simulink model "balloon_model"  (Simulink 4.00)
settings: Solver=ode45  StartTime=0.0  StopTime=5000  RelTol=1e-3
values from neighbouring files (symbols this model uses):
  C = V*rho_a*c_a    [balloon_init.m]
  f = f / 10    [balloon_init.m]
  g = 9.80665    [balloon_init.m]
  m = input('Inserire le prime due cifre (esclusi zeri) del proprio numero di matricola:\n\n')    [balloon_init.m]
  rho_a = 1.2928    [balloon_init.m]
  Ta = 20+273.15    (= 293.15)    [balloon_init.m]
  theta_t = theta_t/50    [balloon_init.m]
  V = V*m*2    [balloon_init.m]
  x1_0 = x1_d    [balloon_init.m]
  x2_0 = 100    [balloon_init.m]
  x3_0 = 0    [balloon_init.m]

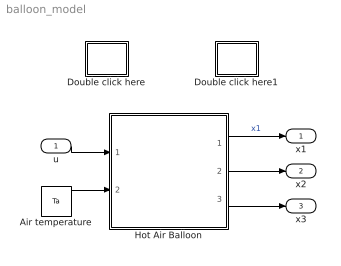
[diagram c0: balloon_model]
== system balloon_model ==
  u : Inport  Port=1  LatchInput=off
  Air temperature : Constant  Value=Ta
  Double click here : Subsystem
  Double click here1 : Subsystem
  Hot Air Balloon : Subsystem  mask{V=V, m=m, C=C, theta_t=theta_t, f=f, g=g}
      mask prompts: V "Balloon's volume (V)"; m "Balloon's total mass (m)"; C "Thermal capacitance (C)"; theta_t "Thermal resistance (theta_t)"; f "Aerodynamic viscous friction (f)"; g "Gravitational acceleration (g)"
  x1 : Outport  Port=1
  x2 : Outport  Port=2
  x3 : Outport  Port=3
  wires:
  u/1 -> Hot Air Balloon/1(u)
  Hot Air Balloon/1(x1) -> x1/1  "x1"
  Hot Air Balloon/2(x2) -> x2/1
  Hot Air Balloon/3(x3) -> x3/1
  Air temperature/1 -> Hot Air Balloon/2(Ta)

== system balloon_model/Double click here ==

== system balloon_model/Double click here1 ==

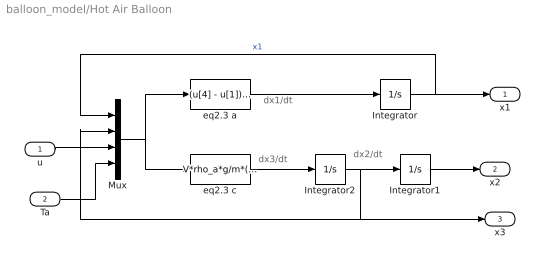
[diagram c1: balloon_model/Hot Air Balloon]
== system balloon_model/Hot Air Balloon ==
  note: dx1/dt
  note: dx3/dt
  note: dx2/dt
  u : Inport  Port=1  LatchInput=off
  Ta : Inport  Port=2  LatchInput=off
  Integrator : Integrator  ExternalReset=none  InitialConditionSource=internal  InitialCondition=x1_0  LimitOutput=off  UpperSaturationLimit=inf  LowerSaturationLimit=-inf  ShowSaturationPort=off  ShowStatePort=off  AbsoluteTolerance=auto
  Integrator1 : Integrator  ExternalReset=none  InitialConditionSource=internal  InitialCondition=x2_0  LimitOutput=off  UpperSaturationLimit=inf  LowerSaturationLimit=0  ShowSaturationPort=off  ShowStatePort=off  AbsoluteTolerance=auto
  Integrator2 : Integrator  ExternalReset=none  InitialConditionSource=internal  InitialCondition=x3_0  LimitOutput=off  UpperSaturationLimit=inf  LowerSaturationLimit=-inf  ShowSaturationPort=off  ShowStatePort=off  AbsoluteTolerance=auto
  Mux : Mux  Inputs=4
  eq2.3 a : Fcn  Expr=(u[4] - u[1])/(C*theta_t) + u[3]/C
  eq2.3 c : Fcn  Expr=V*rho_a*g/m*(1 - u[4]/u[1]) - f/m*u[2] - g
  x1 : Outport  Port=1
  x2 : Outport  Port=2
  x3 : Outport  Port=3
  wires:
  eq2.3 a/1 -> Integrator/1
  eq2.3 c/1 -> Integrator2/1
  Mux/1 -> eq2.3 a/1, eq2.3 c/1
  Integrator/1 -> Mux/1, x1/1  "x1"
  Integrator2/1 -> Integrator1/1, x3/1, Mux/2
  Integrator1/1 -> x2/1
  u/1 -> Mux/3
  Ta/1 -> Mux/4
